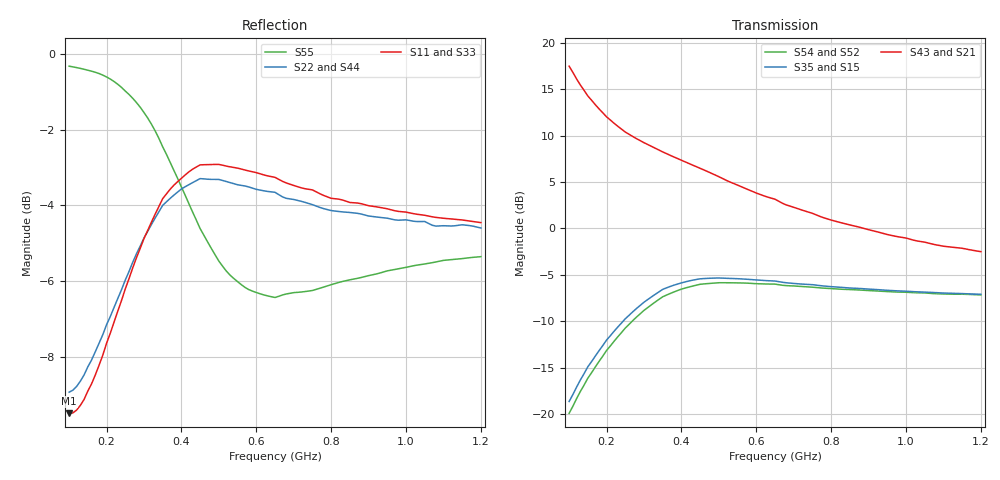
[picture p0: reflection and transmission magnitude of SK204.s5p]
!  POLYFET RF DEVICES
!  S PARAMETERS FOR
!  SK204 (EACH SIDE)
!  VDS=28, IDQ=800MA
! Date: Thu Sep 24 15:21:25 1998
! S2A 4Die, AP pkg, Vds=28Vdc, Idq=800ma, Vgsth=3.48Vdc
!AWR Design Environment (2053) Wed Feb 04 15:23:40 2004
!freq-unit  param-type  data-format  keyword  impedance-ohms
# MHz  S  MA  R  50
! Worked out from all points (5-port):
!   111 points, 100 MHz to 1.2 GHz, reference 50 ohm
!   strongest paths, dB at 100 MHz, 370 MHz, 650 MHz, 930 MHz, 1.2 GHz:
!     S43: 17.5, 7.9, 3.1, -0.4, -2.5
!     S21: 17.5, 7.9, 3.1, -0.4, -2.5
!     S35: -18.6, -6.2, -5.7, -6.6, -7.1
!     S15: -18.6, -6.2, -5.7, -6.6, -7.1
!     S54: -19.9, -7.0, -6.0, -6.7, -7.2
!     S52: -19.9, -7.0, -6.0, -6.7, -7.2
!   lowest |S11| = -9.5 dB at 100 MHz (marker M1), VSWR 2.01, Z = 51.9 - j36.2 ohm
!   |S11| at or under -10 dB: nowhere
